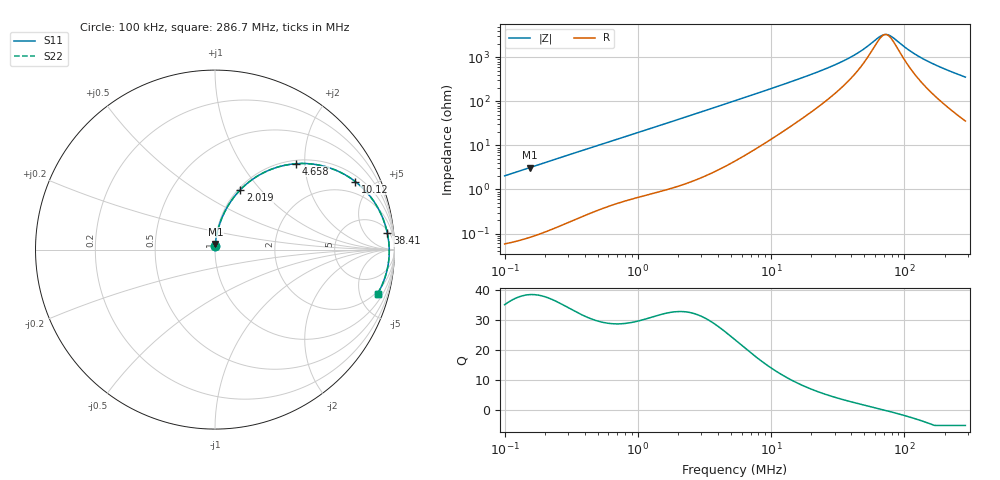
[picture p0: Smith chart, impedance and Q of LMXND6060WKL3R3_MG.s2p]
! LMXND6060WKL3R3_MG  S-PARAMETER MODEL  ( General Type )
! Model Generated by TAIYO YUDEN Corporation (http://www.ty-top.com)
! Version 1.0
! TAIYO YUDEN Control No. 191025NI43SB-FBB
! Copyright(c) 2019 TAIYO YUDEN CO.,LTD. All Rights Reserved.
! Product Description (link to TY-COMPAS)
! https://ds.yuden.co.jp/TYCOMPAS/or/detail?pn=LMXND6060WKL3R3NMG&u=M
! Products Name : Inductors
! Characteristics :
!  Inductance : 3.3 uH , SRF(min) : 55 MHz , DC Resistance(max) : 0.048 Ohm
!  Rated Current : Saturation :2800 mA , Temp Rise : 2750 mA
!  Case Size : 6.0 x 6.0 / 0.236 x 0.236 [mm/inch] , Thickness : 2 / 0.079 [mm/inch]
!  (Conditions: Temperature = 25 degC , DC Bias Current/Voltage = 0A / 0V)
! External Node Assignments :
!  1  o---GGG---o  2
! GND o---------o GND
! Frequency Range : 0.1MHz  -  286.687601MHz  [ 402 STEP ]
# MHz S RI R 50
! Freq[MHz].  S11 Real  S11 Imag  S21 Real  S21 Imag  S12 Real  S12 Imag  S22 Real  S22 Imag
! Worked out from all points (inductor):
!   401 points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, 100 kHz to 286.7 MHz, reference 50 ohm
!   read as one part in series: L = 3.24 uH near 104.1 kHz
!   highest Q = 38.5 at 154.9 kHz (marker M1), where L = 3.24 uH
!   self-resonance near 72.11 MHz
!   S11 on the Smith chart (normalised r, x): 100 kHz: 1.00, +0.04; 2.019 MHz: 1.02, +0.79; 4.658 MHz: 1.07, +1.81; 10.12 MHz: 1.28, +3.97; 38.41 MHz: 7, +18; 286.7 MHz: 1.72, -7.12
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0.1  0.000994 0.0204  0.999 -0.0204  0.999 -0.0204  0.000994 0.0204
0.154938  0.00181 0.0315  0.9982 -0.0315  0.9982 -0.0315  0.00181 0.0315
0.379416  0.00815 0.0756  0.9918 -0.0756  0.9918 -0.0756  0.00815 0.0756
0.761446  0.027 0.1458  0.973 -0.1458  0.973 -0.1458  0.027 0.1458
1.439567  0.0801 0.2562  0.9199 -0.2562  0.9199 -0.2562  0.0801 0.2562
2.019165  0.1411 0.3332  0.8589 -0.3332  0.8589 -0.3332  0.1411 0.3332
3.006369  0.2607 0.4233  0.7393 -0.4233  0.7393 -0.4233  0.2607 0.4233
4.658003  0.452 0.4786  0.548 -0.4786  0.548 -0.4786  0.452 0.4786
5.354322  0.5192 0.4788  0.4808 -0.4788  0.4808 -0.4788  0.5192 0.4788
7.074793  0.6481 0.4521  0.3519 -0.4521  0.3519 -0.4521  0.6481 0.4521
10.12272  0.7822 0.3785  0.2178 -0.3785  0.2178 -0.3785  0.7822 0.3785
13.91854  0.8628 0.299  0.1372 -0.299  0.1372 -0.299  0.8628 0.299
20.31517  0.9195 0.2095  0.0805 -0.2095  0.0805 -0.2095  0.9195 0.2095
38.40725  0.9603 0.0911  0.0397 -0.0911  0.0397 -0.0911  0.9603 0.0911
48.76805  0.9665 0.055  0.0335 -0.055  0.0335 -0.055  0.9665 0.055
67.05509  0.9705 0.0101  0.0295 -0.0101  0.0295 -0.0101  0.9705 0.0101
72.61158  0.9709 -0.000971  0.0291 0.000971  0.0291 0.000971  0.9709 -0.000971
77.07906  0.9709 -0.00929  0.0291 0.00929  0.0291 0.00929  0.9709 -0.00929
110.2859  0.968 -0.0611  0.032 0.0611  0.032 0.0611  0.968 -0.0611
137.2773  0.9626 -0.0959  0.0374 0.0959  0.0374 0.0959  0.9626 -0.0959
192.5478  0.9463 -0.1575  0.0537 0.1575  0.0537 0.1575  0.9463 -0.1575
286.6876  0.9064 -0.2452  0.0936 0.2452  0.0936 0.2452  0.9064 -0.2452
